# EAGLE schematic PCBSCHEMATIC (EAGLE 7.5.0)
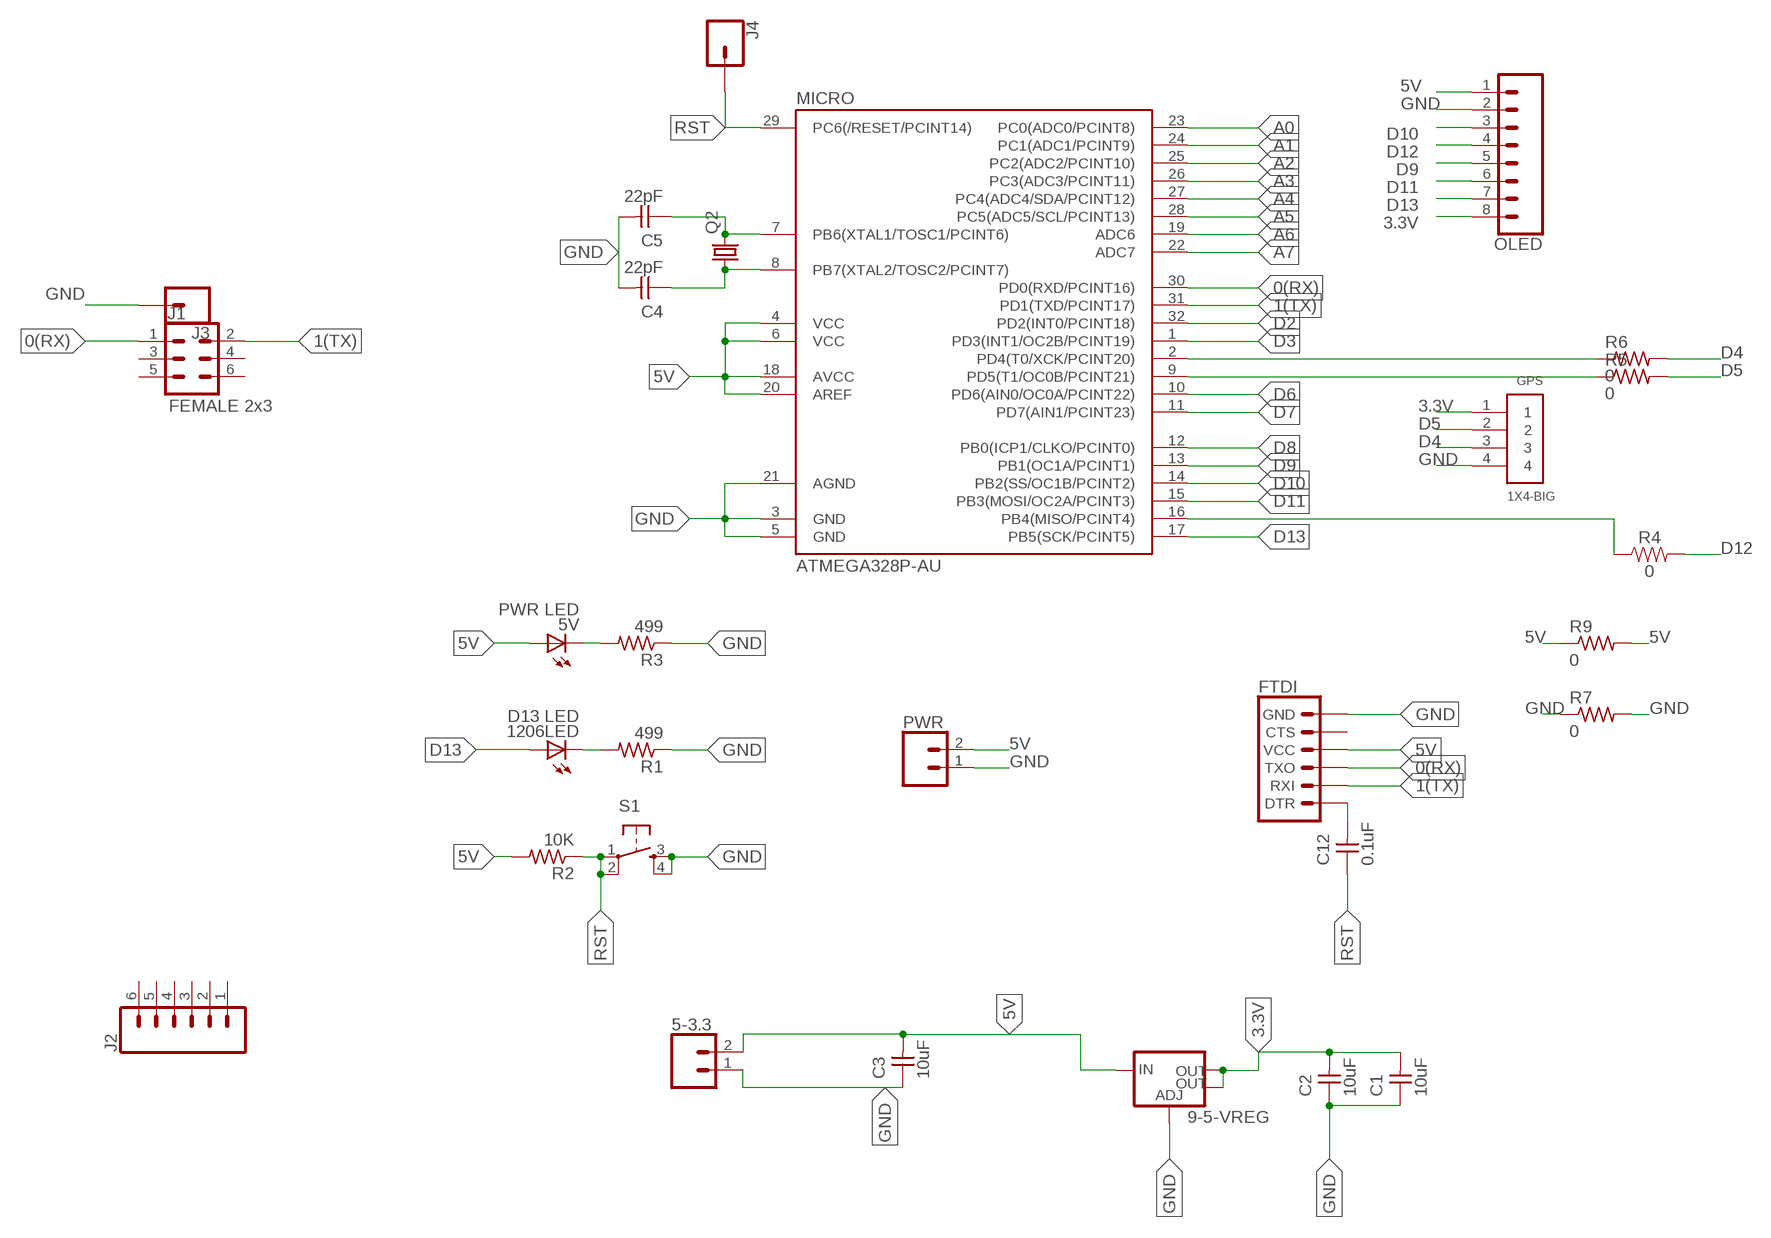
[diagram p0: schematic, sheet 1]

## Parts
5-3.3  CONN_02LOCK  [1X02_LOCK]
5V  PWR LED  LEDFAB1206  [LED1206FAB]
9-5-VREG  V_REG_LM1117SOT223  [SOT223]
1206LED  D13 LED  LEDFAB1206  [LED1206FAB]
C1  10uF  CAP-UNPOLARIZEDFAB  [C1206FAB]
C2  10uF  CAP-UNPOLARIZEDFAB  [C1206FAB]
C3  10uF  CAP-UNPOLARIZEDFAB  [C1206FAB]
C4  22pF  CAP-UNPOLARIZEDFAB  [C1206FAB]
C5  22pF  CAP-UNPOLARIZEDFAB  [C1206FAB]
C12  0.1uF  CAP-UNPOLARIZEDFAB  [C1206FAB]
FTDI  6_PIN_SERIAL_TARGET_SILK  [1X06]
GPS  1X4-BIG  [1X04-BIG]
J1  FEMALE 2x3  CONN_03X2FEMALE  [2X3]
J2  CONN_06SILK_FEMALE_PTH  [1X06]
J3  CONN_01  [1X01]
J4  CONN_01  [1X01]
MICRO  ATMEGA328P-AU  ATMEGA48/88/168-AU  [TQFP32-08]
OLED  CONN_08"  [1X08]
PWR  CONN_02LOCK  [1X02_LOCK]
Q2  CRYSTALHC49U70  [HC49U70]
R1  499  RES-US1206FAB  [R1206FAB]
R2  10K  RES-US1206FAB  [R1206FAB]
R3  499  RES-US1206FAB  [R1206FAB]
R4  0  10MOHM-HORIZ-1/4W-5%  [AXIAL-0.3]
R5  0  R-US_0207/12  [0207/12]
R6  0  R-US_0207/12  [0207/12]
R7  0  RES-US1206FAB  [R1206FAB]
R9  0  R-US_0207/12  [0207/12]
S1  6MM_SWITCH6MM_SWITCH  [6MM_SWITCH]

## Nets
0(RX): FTDI.3(TXO) J1.1 MICRO.30(PD0(RXD/PCINT16))
1(TX): FTDI.2(RXI) J1.2 MICRO.31(PD1(TXD/PCINT17))
3.3V: 9-5-VREG.2(OUT) 9-5-VREG.4(OUT) C1.2 C2.2 GPS.1 OLED.8
5V: 5-3.3.2 5V.1(A) 9-5-VREG.3(IN) C3.2 FTDI.4(VCC) MICRO.4(VCC) MICRO.6(VCC) MICRO.18(AVCC) MICRO.20(AREF) OLED.1 PWR.2 R2.2 R9.1 R9.2
A0: MICRO.23(PC0(ADC0/PCINT8))
A1: MICRO.24(PC1(ADC1/PCINT9))
A2: MICRO.25(PC2(ADC2/PCINT10))
A3: MICRO.26(PC3(ADC3/PCINT11))
A4: MICRO.27(PC4(ADC4/SDA/PCINT12))
A5: MICRO.28(PC5(ADC5/SCL/PCINT13))
A6: MICRO.19(ADC6)
A7: MICRO.22(ADC7)
D2: MICRO.32(PD2(INT0/PCINT18))
D3: MICRO.1(PD3(INT1/OC2B/PCINT19))
D4: GPS.3 R6.2
D5: GPS.2 R5.2
D6: MICRO.10(PD6(AIN0/OC0A/PCINT22))
D7: MICRO.11(PD7(AIN1/PCINT23))
D8: MICRO.12(PB0(ICP1/CLKO/PCINT0))
D9: MICRO.13(PB1(OC1A/PCINT1)) OLED.5
D10: MICRO.14(PB2(SS/OC1B/PCINT2)) OLED.3
D11: MICRO.15(PB3(MOSI/OC2A/PCINT3)) OLED.6
D12: OLED.4 R4.P$2
D13: 1206LED.1(A) MICRO.17(PB5(SCK/PCINT5)) OLED.7
GND: 5-3.3.1 9-5-VREG.1(ADJ) C1.1 C2.1 C3.1 C4.2 C5.2 FTDI.6(GND) GPS.4 J3.1 MICRO.3(GND) MICRO.5(GND) MICRO.21(AGND) OLED.2 PWR.1 R1.1 R3.1 R7.1 R7.2 S1.3(S) S1.4(S1)
N$1: 1206LED.2(C) R1.2
N$2: 5V.2(C) R3.2
N$3: C5.1 MICRO.7(PB6(XTAL1/TOSC1/PCINT6)) Q2.2
N$4: C4.1 MICRO.8(PB7(XTAL2/TOSC2/PCINT7)) Q2.1
N$6: MICRO.16(PB4(MISO/PCINT4)) R4.P$1
N$7: MICRO.9(PD5(T1/OC0B/PCINT21)) R5.1
N$8: MICRO.2(PD4(T0/XCK/PCINT20)) R6.1
N$16: C12.2 FTDI.1(DTR)
RST: C12.1 J4.1 MICRO.29(PC6(/RESET/PCINT14)) R2.1 S1.1(P) S1.2(P1)
Unconnected: FTDI.5(CTS) J1.3 J1.4 J1.5 J1.6 J2.1 J2.2 J2.3 J2.4 J2.5 J2.6

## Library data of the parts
5-3.3 PWR = SparkFun-Connectors:CONN_02: Multi connection point. Often used as Generic Header-pin footprint for 0.1 inch spaced/style header connections
5V 1206LED = fab:LED: LED
9-5-VREG = fab:V_REG_LM1117: Voltage Regulator LM1117 Standard adjustable voltage regulator but in SMD form. Spark Fun Electronics SKU : COM-00595; PROD_ID: VREG-08170
C1-C5 C12 = fab:CAP-UNPOLARIZED
FTDI = SparkFun-Connectors:6_PIN_SERIAL_TARGET: 6-pin header connection for use with the "FTDI BASIC" pinout - TARGET SIDE. Also known as "Arduino Serial Program Header". It is used to mate with our FTDI Basic serial programmers using the Arduino IDE. Note, this device has "TARGET" in the name. It is intended to be used on a design that contains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
GPS = adafruit:1X4: 4-pin connector
J1 = SparkFun-Connectors:CONN_03X2: Multi connection point. Often used as Generic Header-pin footprint for 0.1 inch spaced/style header connections You can populate with any combo of single row headers, but if you'd like an exact match, check these: Header - 2x3 (Male, 0.1") (PRT-12807) Header - 2x3 (Female, 0.1") (PRT-13010) 2x3 Pin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; PROD_ID: CONN-11566
J2 = SparkFun-Connectors:CONN_06: Multi connection point. Often used as Generic Header-pin footprint for 0.1 inch spaced/style header connections On any of the 0.1 inch spaced packages, you can populate with these: Break Away Headers - Straight (PRT-00116) Break Away Male Headers - Right Angle (PRT-00553) Female Headers (PRT-00115)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; PROD_ID: CONN-08437
J3 J4 = SparkFun-Connectors:CONN_01: Single connection point. Often used as Generic Header-pin footprint for 0.1 inch spaced/style header connections
MICRO = atmega8:ATMEGA48/88/168
OLED = SparkFun-Connectors:CONN_08: Multi connection point. Often used as Generic Header-pin footprint for 0.1 inch spaced/style header connections On any of the 0.1 inch spaced packages, you can populate with these: Break Away Headers - Straight (PRT-00116) Break Away Male Headers - Right Angle (PRT-00553) Female Headers (PRT-00115)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; PROD_ID: CONN-08438
Q2 = crystal:CRYSTAL: CRYSTAL; OC_FARNELL: unknown; OC_NEWARK: unknown
R1-R3 R7 = fab:RES-US: Resistor (US Symbol)
R4 = SparkFun-Resistors:10MOHM: RES-09327; PROD_ID: RES-09327; VALUE: 10M
R5 R6 R9 = adafruit:R-US_: RESISTOR, American symbol
S1 = fab:6MM_SWITCH: OMRON SWITCH

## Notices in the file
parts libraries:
SparkFun-Connectors: Licensing: Creative Commons ShareAlike 4.0 International - https://creativecommons.org/licenses/by-sa/4.0
